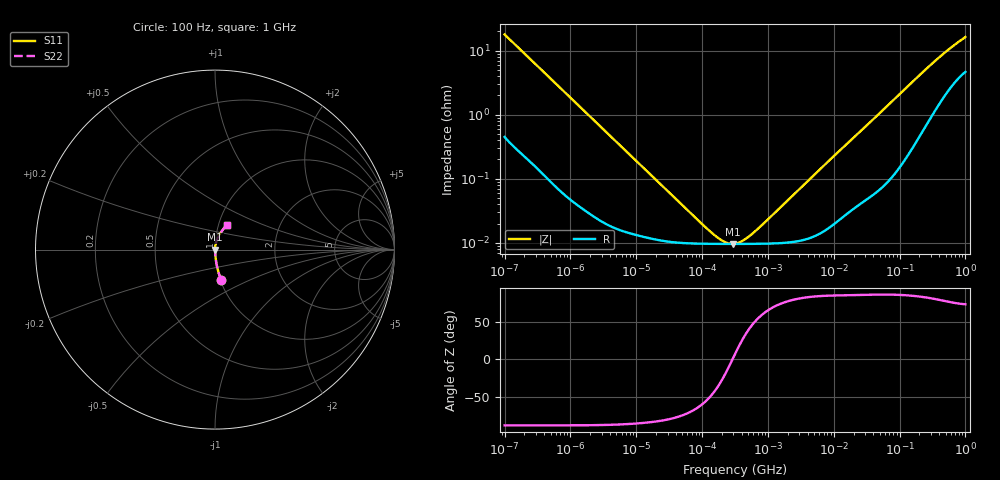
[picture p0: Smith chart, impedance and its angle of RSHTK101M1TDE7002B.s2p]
! RSHTK101M1TDE7002B  S-PARAMETER MODEL  (General Type)
! Model Generated by ELNA Corporation (http://www.ty-top.com)
! Version 1.0
! ELNA Control No.240315
! Copyright (c) 2024 ELNA CO.,LTD. All Rights Reserved.
! Products Name : CONDUCTIVE POLYMER HYBRID ALUMINUM ELECTROLYTIC CAPACITORS
! Characteristics :
!  Capacitance  :  100uF  ,  Rated voltage  :  25V
!  Operating Temp. Range  :  -55 to +125 degC  ,  Endurance  :  6000hr at 125 degC
!  Dimension D  :  6.3mm  ,  Dimension L  :  7.7mm
! Frequency Range : 100Hz - 1GHz
! External Node Assignments :
!  1  o---| |---o  2
# MHz S RI R 50
!Freq[MHz].  S11 Real  S11 Imag  S21 Real  S21 Imag  S12 Real  S12 Imag  S22 Real  S22 Imag
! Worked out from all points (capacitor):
!   401 points, 100 Hz to 1 GHz, reference 50 ohm
!   read as one part in series: C = 88.7 uF near 108 Hz
!   lowest |Z| = 9.61 mohm at 291.7 kHz (marker M1)
!   series resonance near 290.3 kHz, so ESL is about 3.4 nH
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0.0001  0.0351 -0.172  0.9649 0.172  0.9649 0.172  0.0351 -0.172
0.000113  0.0282 -0.1537  0.9718 0.1537  0.9718 0.1537  0.0282 -0.1537
0.000183  0.0119 -0.097  0.9881 0.097  0.9881 0.097  0.0119 -0.097
0.000309  0.00489 -0.0584  0.9951 0.0584  0.9951 0.0584  0.00489 -0.0584
0.000613  0.00162 -0.0298  0.9984 0.0298  0.9984 0.0298  0.00162 -0.0298
0.001488  0.000501 -0.0124  0.9995 0.0124  0.9995 0.0124  0.000501 -0.0124
0.022131  0.000111 -0.000862  0.9999 0.000862  0.9999 0.000862  0.000111 -0.000862
0.094406  9.69e-05 -0.000183  0.9999 0.000183  0.9999 0.000183  9.69e-05 -0.000183
0.153109  9.63e-05 -9.13e-05  0.9999 9.13e-05  0.9999 9.13e-05  9.63e-05 -9.13e-05
0.220039  9.61e-05 -3.74e-05  0.9999 3.74e-05  0.9999 3.74e-05  9.61e-05 -3.74e-05
0.291743  9.6e-05 6.85e-07  0.9999 -6.85e-07  0.9999 -6.85e-07  9.6e-05 6.85e-07
0.316228  9.6e-05 1.15e-05  0.9999 -1.15e-05  0.9999 -1.15e-05  9.6e-05 1.15e-05
0.356862  9.61e-05 2.78e-05  0.9999 -2.78e-05  0.9999 -2.78e-05  9.61e-05 2.78e-05
0.402717  9.61e-05 4.45e-05  0.9999 -4.45e-05  0.9999 -4.45e-05  9.61e-05 4.45e-05
0.60256  9.63e-05 0.000106  0.9999 -0.000106  0.9999 -0.000106  9.63e-05 0.000106
1.017419  9.72e-05 0.000215  0.9999 -0.000215  0.9999 -0.000215  9.72e-05 0.000215
4.704354  0.000123 0.00107  0.9999 -0.00107  0.9999 -0.00107  0.000123 0.00107
69.9842  0.00117 0.0147  0.9988 -0.0147  0.9988 -0.0147  0.00117 0.0147
169.8244  0.00463 0.0348  0.9954 -0.0348  0.9954 -0.0348  0.00463 0.0348
365.1741  0.0174 0.0694  0.9826 -0.0694  0.9826 -0.0694  0.0174 0.0694
641.9482  0.04 0.1059  0.96 -0.1059  0.96 -0.1059  0.04 0.1059
1000  0.0656 0.1398  0.9344 -0.1398  0.9344 -0.1398  0.0656 0.1398
